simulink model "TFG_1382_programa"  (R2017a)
settings: Solver=FixedStepAuto  StartTime=0.0  StopTime=inf  RelTol=1e-3  EnableMultiTasking=on
libraries: arduinolib x3, simulink x2

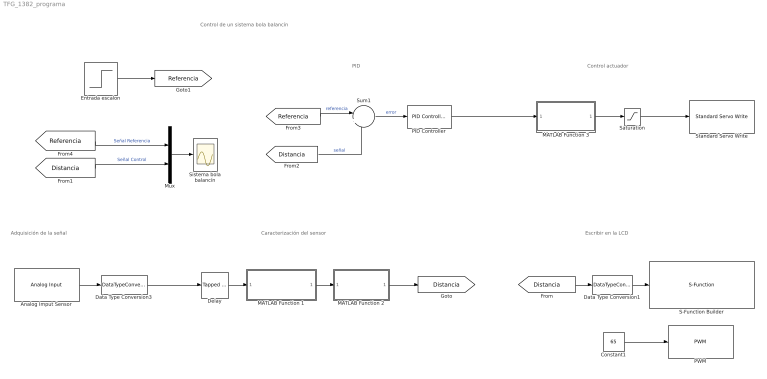
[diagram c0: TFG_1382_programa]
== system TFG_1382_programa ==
  note: Control de un sistema bola balancín
  note: Control actuador
  note: PID
  note: Escribir en la LCD
  note: Adquisición de la señal
  note: Caracterización del sensor
  Analog Imput Sensor : arduinolib/Analog Input  pinNumber=0  sampleTime=-1  blockPlatform=arduino
  Constant1 : Constant  Value=65
  Data Type Conversion1 : DataTypeConversion  OutDataTypeStr=uint16
  Data Type Conversion3 : DataTypeConversion  OutDataTypeStr=double
  Delay : simulink/Discrete/Tapped Delay  vinit=0.0  samptime=-1  NumDelays=20  DelayOrder=Oldest  includeCurrent=off
  Entrada escalon : Step  After=33
  MATLAB Function 1 : MATLAB Function  TreatAsAtomicUnit=on
  MATLAB Function 2 : MATLAB Function  TreatAsAtomicUnit=on
  MATLAB Function 3 : MATLAB Function  TreatAsAtomicUnit=on
  Mux : Mux  Inputs=2
  PID Controller : simulink/Continuous/PID Controller  Controller=PID  TimeDomain=Discrete-time  SampleTime=0.01  IntegratorMethod=Forward Euler  FilterMethod=Forward Euler  Form=Parallel  UseFilter=off  ControllerParametersSource=internal  P=2  I=0.4  D=2.2  N=100  InitialConditionSource=internal  InitialConditionForIntegrator=0  InitialConditionForFilter=0  ExternalReset=none  LimitOutput=off  UpperSaturationLimit=inf  LowerSaturationLimit=-inf  LinearizeAsGain=off  AntiWindupMode=none  Kb=1  TrackingMode=off  Kt=1  PParamMin=[]  PParamMax=[]  IParamMin=[]  IParamMax=[]  DParamMin=[]  DParamMax=[]  NParamMin=[]  NParamMax=[]  KbParamMin=[]  KbParamMax=[]  KtParamMin=[]  KtParamMax=[]  POutMin=[]  POutMax=[]  IOutMin=[]  IOutMax=[]  DOutMin=[]  DOutMax=[]  NOutMin=[]  NOutMax=[]  KbOutMin=[]  KbOutMax=[]  KtOutMin=[]  KtOutMax=[]  IntegratorOutMin=[]  IntegratorOutMax=[]  FilterOutMin=[]  FilterOutMax=[]  SumOutMin=[]  SumOutMax=[]  SumI1OutMin=[]  SumI1OutMax=[]  SumI2OutMin=[]  SumI2OutMax=[]  SumI3OutMin=[]  SumI3OutMax=[]  SumDOutMin=[]  SumDOutMax=[]  SaturationOutMin=[]  SaturationOutMax=[]  IntegratorContinuousStateAttributes=''  IntegratorStateMustResolveToSignalObject=off  IntegratorRTWStateStorageClass=Auto  FilterContinuousStateAttributes=''  FilterStateMustResolveToSignalObject=off  FilterRTWStateStorageClass=Auto  DifferentiatorICPrevScaledInput=0  DifferentiatorOutMin=[]  DifferentiatorOutMax=[]  InitialConditionSetting=State (most efficient)
  PWM : arduinolib/PWM  pinNumber=9  blockPlatform=arduino
  S-Function Builder : S-Function  InitFcn=try, set_param(gcb,'FunctionName','Lcd'), end  FunctionName=Lcd  SFunctionModules=Lcd_wrapper  SFunctionDeploymentMode=off  EnableBusSupport=off
  Saturation : Saturate  UpperLimit=180  LowerLimit=0
  Sistema bola balancín : Scope
  Standard Servo Write : arduinolib/Standard Servo Write  pinNumber=7  blockPlatform=arduino
  Sum1 : Sum  Inputs=|+-
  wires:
  MATLAB Function 3/1(grados) -> Saturation/1
  Constant1/1 -> PWM/1
  Data Type Conversion1/1 -> S-Function Builder/1
  MATLAB Function 1/1(sensorfilter) -> MATLAB Function 2/1(posv)
  Data Type Conversion3/1 -> Delay/1
  Sum1/1 -> PID Controller/1  "error"
  Analog Imput Sensor/1 -> Data Type Conversion3/1
  Delay/1 -> MATLAB Function 1/1(sensor)
  MATLAB Function 2/1(poscm) -> [Distancia]
  [Distancia] -> Data Type Conversion1/1
  [Distancia] -> Sum1/2  "señal"
  Mux/1 -> Sistema bola balancín/1
  [Distancia] -> Mux/2  "Señal Control"
  [Referencia] -> Mux/1  "Señal Referencia"
  PID Controller/1 -> MATLAB Function 3/1(pid)
  Entrada escalon/1 -> [Referencia]
  [Referencia] -> Sum1/1  "referencia"
  Saturation/1 -> Standard Servo Write/1

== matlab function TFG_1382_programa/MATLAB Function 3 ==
function grados = fcn(pid)

 grados = ((pid - (-180))*(180 - 0))/(180 - (-180)) + 0;
 
end

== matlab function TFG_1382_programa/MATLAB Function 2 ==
function poscm = funcion(posv)

poscm=-0.1138*posv+77.958;

end

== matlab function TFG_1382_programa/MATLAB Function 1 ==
function sensorfilter = filter(sensor)
sensorfilter=0.0;
%%sortedValues=[0,0,0,0,0,0,0,0,0,0,0,0,0,0,0];
sortedValues=[0,0,0,0,0,0,0,0,0,0,0,0,0,0,0,0,0,0,0,0];
for a=1:20 % medidas
    if(sensor(a)<sortedValues(1) || a==1)
        j=1; %%inserta en la primera posicion
    else
      for j=2:a
          if(sortedValues(j-1)<=sensor(a)&& sortedValues(j)>=sensor(a))
          %%j is insert position
          break;
          end
      end
    end
    for k=a:-1:j+1 %movemos los valores una posición
        sortedValues(k)=sortedValues(k-1);
    end
    sortedValues(j)=sensor(a); %se inserta lectura actual
end
for a=8:12 %hacemos media de los intermedios
    sensorfilter=sensorfilter+sortedValues(a);
end
sensorfilter=sensorfilter/5;
end
